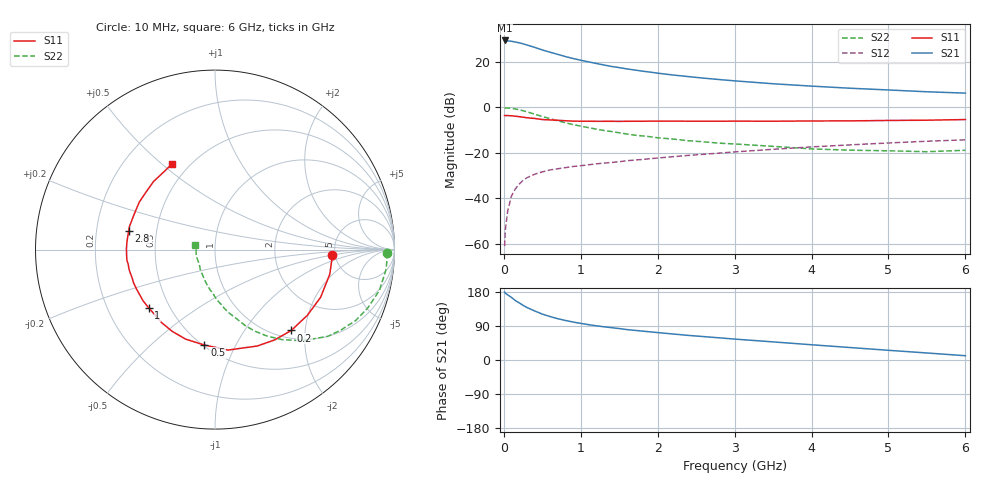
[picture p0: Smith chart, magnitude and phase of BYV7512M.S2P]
! SIEMENS Small Signal Semiconductors
! BFY420
! Si NPN RF SIEGET Grounded Emitter Transistor in MICRO-X
! VCE = 0.75 V  IC = 12 mA
! Common Emitter S-Parameters:  October  1996
# GHz  S  MA  R  50
!  f  S11  S21  S12  S22
! GHz  MAG  ANG  MAG  ANG  MAG  ANG  MAG  ANG
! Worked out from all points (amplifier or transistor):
!   36 points, 10 MHz to 6 GHz, reference 50 ohm
!   highest |S21| = 29.2 dB at 10 MHz (marker M1)
!   |S21| within 3 dB of that: start of sweep to 398.5 MHz
!   unconditionally stable (mu >= 1): 2.182 GHz to end of sweep
!   at 250 MHz: K = 0.23, MSG = 29.9 dB, |S12| = -32.1 dB
!   at 1.4 GHz: K = 0.83, MSG = 21.0 dB, |S12| = -24.3 dB
!   at 6 GHz: K = 1.11, MAG = 8.2 dB, |S12| = -14.3 dB
!   S11 on the Smith chart (normalised r, x): 10 MHz: 4.72, -0.53; 200 MHz: 1.15, -1.69; 500 MHz: 0.51, -0.76; 1 GHz: 0.38, -0.33; 2.8 GHz: 0.34, +0.09; 6 GHz: 0.41, +0.54
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0.01  0.6541 -2.8  28.91 179.3  0.0009 94.3  0.96 -1.1
0.02  0.6533 -5.1  28.79 176.3  0.0021 96.8  0.9607 -2.6
0.1  0.6458 -24.3  27.73 165.0  0.0114 79.9  0.9437 -14.0
0.15  0.6315 -35.5  26.71 156.8  0.0162 73.6  0.9116 -20.8
0.2  0.6193 -46.7  25.71 150.8  0.0206 70.0  0.8775 -26.8
0.25  0.6029 -56.6  24.38 144.2  0.0248 65.0  0.8323 -32.6
0.3  0.5865 -66.3  23.01 138.6  0.0284 62.2  0.7924 -37.6
0.4  0.5645 -82.6  20.43 129.5  0.0339 57.2  0.7026 -46.3
0.5  0.535 -96.3  17.91 121.1  0.0382 53.1  0.6246 -53.4
0.6  0.525 -108.1  15.98 114.7  0.0421 50.3  0.5596 -59.2
0.7  0.5142 -117.6  14.34 109.0  0.0446 48.7  0.5039 -64.1
0.8  0.504 -126.2  12.83 104.3  0.0473 47.3  0.4556 -68.3
1  0.4917 -138.6  10.66 96.6  0.0521 46.3  0.3834 -74.8
1.1  0.4919 -144.6  9.835 93.3  0.0546 46.0  0.3557 -78.3
1.4  0.4901 -157.8  7.792 85.3  0.0613 45.7  0.292 -85.9
1.6  0.49 -164.9  6.878 80.3  0.067 45.3  0.258 -90.8
2.2  0.4934 179.6  5.055 68.6  0.0822 44.8  0.1997 -102.9
2.8  0.4918 167.8  4.027 58.5  0.0984 42.7  0.1625 -114.2
3.5  0.4918 155.9  3.254 47.8  0.1192 39.0  0.1383 -126.3
4.5  0.5002 140.3  2.598 32.9  0.1491 31.5  0.1141 -145.1
5.5  0.5177 123.9  2.172 18.5  0.179 22.3  0.1055 -177.9
6  0.5349 116.4  2.029 11.3  0.1925 17.6  0.1136 165.8
